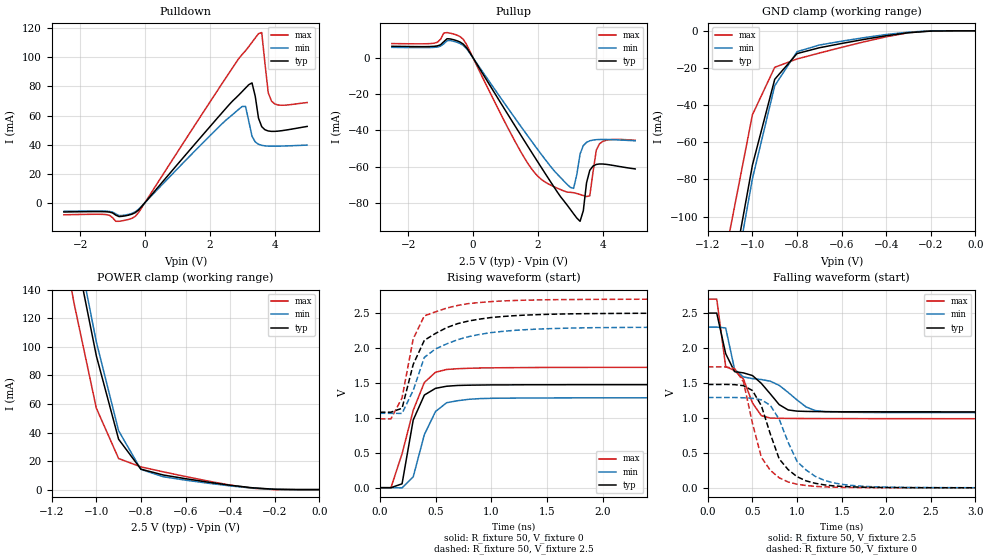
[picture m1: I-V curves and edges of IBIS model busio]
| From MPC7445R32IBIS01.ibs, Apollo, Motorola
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| *   busio Model   *
[Model]   busio
Model_type   I/O
Polarity   Non-Inverting
Vinl = 0.5V
Vinh = 1.7V
Vmeas = 1.25V
Cref = 0
Rref = 50
Vref = 1.25V
|   typ   min   max
C_comp   3.129162e-12   2.489012e-12   3.347377e-12
|   typ   min   max
[Voltage range]   2.5V   2.3V   2.7V
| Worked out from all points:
|   slope of the pulldown table from 0 to 0.375 V, typ, clamps not added: 37.9 ohm
|   slope of the pullup table from 0 to 0.375 V, typ, clamps not added: 34.1 ohm
|   GND clamp passes 1 mA (typ) near -0.30 V on its own axis
|   POWER clamp passes 1 mA (typ) near -0.27 V on its own axis
|   falling waveform, R_fixture 50, V_fixture 2.5: 20-80 % time 538ps typ, 710ps min, 331ps max; typ from 2.5 V to 1.08 V
|   rising waveform, R_fixture 50, V_fixture 0: 20-80 % time 133ps typ, 166ps min, 198ps max; typ from 0.001 V to 1.48 V
|   falling waveform, R_fixture 50, V_fixture 0: 20-80 % time 281ps typ, 325ps min, 227ps max; typ from 1.48 V to 0.001 V
|   rising waveform, R_fixture 50, V_fixture 2.5: 20-80 % time 272ps typ, 317ps min, 163ps max; typ from 1.08 V to 2.5 V
[Pulldown]
|   Voltage   I(typ)   I(min)   I(max)
-2.5V     -6.427mA   -5.962mA   -8.362mA
-1.2V     -6.287mA   -5.874mA   -8.227mA
-900mV    -8.603mA   -7.76mA    -12.86mA
-300mV    -6.906mA   -6.35mA    -9.478mA
3V        76.59mA    66.26mA    102.1mA
3.1V      78.93mA    66.3mA     104.6mA
3.3V      82.48mA    45.78mA    110.5mA
3.5V      58.21mA    40.2mA     116.4mA
3.6V      52.32mA    39.46mA    117.1mA
3.8V      49.36mA    38.95mA    75.73mA
3.9V      49.09mA    38.89mA    69.96mA
5V        52.5mA     39.64mA    68.95mA
[GND_clamp]
-2.5V     -1.288A    -1.297A    -1.281A
-1.1V     -138.6mA   -146.9mA   -106.9mA
-1V       -72.27mA   -79.58mA   -45.17mA
-900mV    -26.1mA    -29.56mA   -19.64mA
-800mV    -12.25mA   -11.23mA   -15.16mA
-700mV    -9.123mA   -7.665mA   -11.97mA
-500mV    -4.632mA   -3.69mA    -5.938mA
-300mV    -1.027mA   -696uA     -1.008mA
-200mV    -154uA     0A         0A
0V        0A         0A         0A
[Pullup]
-2.5V     6.34mA     5.759mA    7.847mA
-800mV    10.52mA    9.437mA    13.92mA
-300mV    7.544mA    6.809mA    10.19mA
1.8V      -51.95mA   -45.91mA   -61.16mA
3V        -83.66mA   -71.49mA   -74.25mA
3.1V      -86.08mA   -72.07mA   -74.46mA
3.3V      -90.24mA   -53.08mA   -75.45mA
3.6V      -62.08mA   -45.81mA   -76.15mA
3.7V      -59.72mA   -45.4mA    -63.03mA
3.8V      -58.86mA   -45.19mA   -50.96mA
3.9V      -58.6mA    -45.1mA    -47.45mA
5V        -61.34mA   -45.81mA   -45.52mA
[POWER_clamp]
-2.5V     1.498A     1.508A     1.476A
-1.2V     258.3mA    269.3mA    217.2mA
-1.1V     172.2mA    182.9mA    130.7mA
-1V       93.8mA     103.6mA    57.12mA
-900mV    35.3mA     41.24mA    21.79mA
-800mV    14.33mA    14.14mA    15.91mA
-700mV    10.25mA    9.021mA    12.46mA
-500mV    5.256mA    4.507mA    6.032mA
-300mV    1.276mA    1.06mA     956.8uA
-200mV    246uA      206.6uA    0A
0V        0A         0A         0A
|   typ   min   max
[Ramp]
dV/dt_r   0.88700/1.18552e-10   0.77527/1.60703e-10   1.03781/1.76259e-10
dV/dt_f   0.85113/5.08006e-10   0.74060/7.20844e-10   1.02847/3.22301e-10
[Falling Waveform]
R_fixture = 50
V_fixture = 2.5
V_fixture_min = 2.3
V_fixture_max = 2.7
| time   V(typ)   V(min)   V(max)
0s        2.5V       2.3V       2.7V
100ps     2.5V       2.3V       2.7V
200ps     1.921V     2.288V     1.736V
300ps     1.663V     1.695V     1.678V
600ps     1.495V     1.55V      1.033V
700ps     1.345V     1.526V     999.3mV
900ps     1.115V     1.366V     993.7mV
1.2ns     1.092V     1.107V     991.8mV
1.5ns     1.089V     1.082V     991.1mV
19.7ns    1.081V     1.066V     985.8mV
[Rising Waveform]
R_fixture = 50
V_fixture = 0
V_fixture_min = 0
V_fixture_max = 0
| time   V(typ)   V(min)   V(max)
0s        559.5uV    533.6uV    496.2uV
100ps     567.7uV    529.1uV    -825.3uV
200ps     55.84mV    -2.04mV    486.2mV
300ps     969.5mV    155.6mV    1.108V
400ps     1.327V     760.5mV    1.507V
500ps     1.423V     1.091V     1.653V
600ps     1.453V     1.217V     1.693V
700ps     1.464V     1.246V     1.704V
1.8ns     1.475V     1.287V     1.722V
19.7ns    1.479V     1.293V     1.73V
[Falling Waveform]
R_fixture = 50
V_fixture = 0
V_fixture_min = 0
V_fixture_max = 0
| time   V(typ)   V(min)   V(max)
0s        1.479V     1.293V     1.73V
300ps     1.477V     1.293V     1.706V
400ps     1.462V     1.289V     1.516V
600ps     1.176V     1.26V      437.3mV
700ps     773.4mV    1.182V     251.9mV
900ps     261.9mV    652.6mV    84.6mV
1ns       160.6mV    379mV      52.58mV
1.2ns     66.63mV    168mV      22.49mV
2.3ns     3.182mV    5.564mV    2.474mV
19.7ns    559.4uV    521.4uV    534.7uV
[Rising Waveform]
R_fixture = 50
V_fixture = 2.5
V_fixture_min = 2.3
V_fixture_max = 2.7
| time   V(typ)   V(min)   V(max)
0s        1.081V     1.066V     985.8mV
100ps     1.081V     1.065V     985.8mV
200ps     1.138V     1.064V     1.286V
300ps     1.765V     1.394V     2.132V
400ps     2.111V     1.866V     2.461V
500ps     2.209V     1.987V     2.518V
700ps     2.35V      2.12V      2.61V
1.1ns     2.451V     2.238V     2.674V
2.7ns     2.498V     2.298V     2.699V
19.7ns    2.499V     2.3V       2.7V
